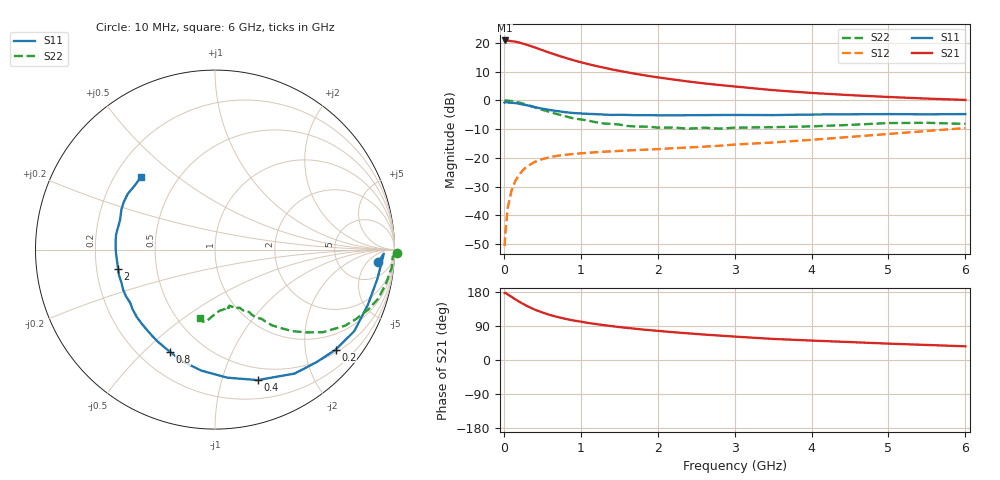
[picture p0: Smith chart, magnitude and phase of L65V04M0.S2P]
!  INFINEON TECHNOLOGIES Small Signal Semiconductors
! BFR380L3 , Si-NPN RF-Transistor in TSLP-3-1
!  Vce=5 V,  Ic=4 mA
! Common Emitter S-Parameters:  07. March 2005
#  GHz  S  MA  R  50
! f  S11  S21  S12  S22
! GHz  Mag  Ang  Mag  Ang  Mag  Ang  Mag  Ang
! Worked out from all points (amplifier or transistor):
!   36 points, 10 MHz to 6 GHz, reference 50 ohm
!   highest |S21| = 20.9 dB at 10 MHz (marker M1)
!   |S21| within 3 dB of that: start of sweep to 462 MHz
!   unconditionally stable (mu >= 1): 2.748 GHz to 4.567 GHz
!   at 250 MHz: K = 0.13, MSG = 22.0 dB, |S12| = -24.3 dB
!   at 1.4 GHz: K = 0.67, MSG = 14.3 dB, |S12| = -17.8 dB
!   at 6 GHz: K = 0.91, MSG = 4.9 dB, |S12| = -9.6 dB
!   S11 on the Smith chart (normalised r, x): 10 MHz: 13, -11; 200 MHz: 0.57, -2.67; 400 MHz: 0.37, -1.31; 800 MHz: 0.32, -0.60; 2 GHz: 0.29, -0.09; 6 GHz: 0.31, +0.38
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0.01  0.9112 -4.4  11.04 176.8  0.0029 77.3  1.013 -1.2
0.02  0.941 -1.4  10.95 177.5  0.005 97.5  0.9909 -2.3
0.05  0.9191 -10.3  10.94 173.1  0.0134 87.3  0.99 -5.7
0.1  0.9056 -20.0  10.72 166.7  0.027 78.9  0.9712 -11.3
0.15  0.8991 -30.4  10.52 160.1  0.0397 74.2  0.9488 -16.8
0.2  0.8737 -39.6  10.15 153.7  0.0509 70.1  0.9168 -21.4
0.3  0.8208 -57.3  9.253 142.5  0.0706 61.7  0.8398 -30.3
0.4  0.7649 -71.9  8.369 133.1  0.0847 54.8  0.7576 -37.4
0.5  0.7168 -84.5  7.49 125.5  0.0949 50.2  0.6868 -42.2
0.6  0.6788 -96.3  6.71 118.7  0.1027 46.4  0.6262 -46.5
0.7  0.6503 -105.6  6.055 113.4  0.1089 44.2  0.5737 -49.8
0.8  0.6223 -113.9  5.502 108.6  0.1129 42.1  0.5283 -53.0
0.9  0.6035 -122.2  5.012 104.5  0.1164 40.7  0.4883 -55.0
1.1  0.5819 -133.7  4.267 97.6  0.1227 39.5  0.4431 -58.7
1.5  0.5604 -152.4  3.269 86.9  0.1321 39.8  0.3796 -64.7
2  0.5505 -168.6  2.515 76.9  0.1418 42.3  0.3353 -71.7
2.2  0.5494 -173.2  2.31 73.4  0.147 43.8  0.3371 -72.3
2.8  0.5561 174.0  1.853 64.5  0.1622 49.0  0.3224 -79.5
3.5  0.5543 162.6  1.506 55.6  0.1851 53.3  0.3417 -85.7
4.5  0.5731 152.8  1.234 47.3  0.2313 59.7  0.3745 -92.8
5.5  0.5724 141.7  1.074 39.7  0.2931 61.6  0.4067 -99.6
6  0.5775 135.3  1.018 36.1  0.3298 61.1  0.39 -102.7
